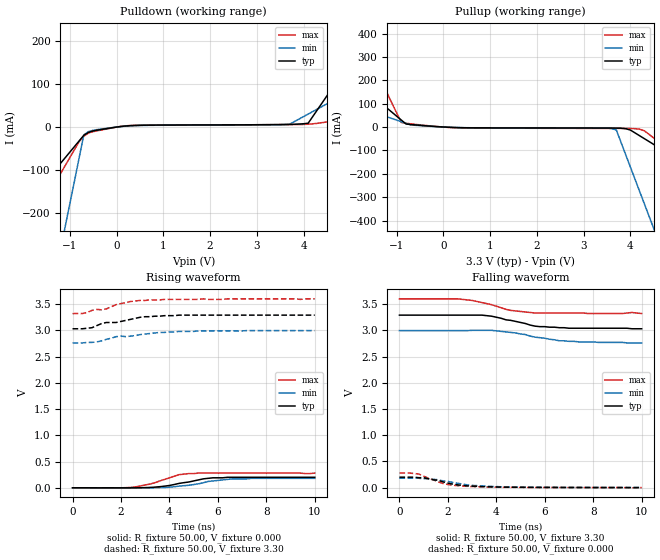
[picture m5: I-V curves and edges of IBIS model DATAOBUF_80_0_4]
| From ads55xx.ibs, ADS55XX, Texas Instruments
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|   Model DATAOBUF_80_0_4
[Model]   DATAOBUF_80_0_4
Model_type   Output
Polarity   Non-Inverting
Vmeas =   1.65V
C_comp   3.00pF   3.00pF   3.00pF
[Temperature Range]   50.00   0.10k   -20.00
[Voltage Range]   3.30V   3.00V   3.60V
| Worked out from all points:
|   slope of the pulldown table from 0 to 0.495 V, typ, clamps not added: 120 ohm
|   slope of the pullup table from 0 to 0.495 V, typ, clamps not added: 147 ohm
|   rising waveform, R_fixture 50.00, V_fixture 0.000: 20-80 % time 1.36ns typ, 1.56ns min, 1.2ns max; typ from 0 V to 0.2 V
|   rising waveform, R_fixture 50.00, V_fixture 3.30: 20-80 % time 1.72ns typ, 2.11ns min, 1.56ns max; typ from 3.03 V to 3.29 V
|   falling waveform, R_fixture 50.00, V_fixture 3.30: 20-80 % time 1.46ns typ, 1.71ns min, 1.42ns max; typ from 3.29 V to 3.03 V
|   falling waveform, R_fixture 50.00, V_fixture 0.000: 20-80 % time 1.35ns typ, 1.57ns min, 1.07ns max; typ from 0.2 V to 0.002 V
[Pulldown]
| voltage   I(typ)   I(min)   I(max)
-3.3V     -359.2mA   -1.41A     -501.7mA
-2.3V     -228.4mA   -874.4mA   -314.5mA
-1.9V     -176.1mA   -660.4mA   -239.6mA
-1.5V     -123.7mA   -446.3mA   -164.7mA
-1V       -58.35mA   -178.7mA   -71.13mA
-700mV    -19.11mA   -18.13mA   -21.33mA
-500mV    -8.95mA    -7.42mA    -10.52mA
300mV     3.33mA     2.8mA      3.59mA
3.7V      6.18mA     6.49mA     5.76mA
4.1V      8.96mA     30.21mA    6.69mA
5.5V      230.9mA    113.2mA    28.31mA
6.6V      405.2mA    178.5mA    46.3mA
[Pullup]
| voltage   I(typ)   I(min)   I(max)
-3.3V     431.1mA    186.7mA    1.012A
-1.9V     197.1mA    91.11mA    432.9mA
-900mV    29.86mA    22.81mA    19mA
-800mV    13.14mA    15.98mA    16.23mA
400mV     -2.71mA    -2.43mA    -3.79mA
3.6V      -4.13mA    -6.27mA    -5.71mA
3.7V      -4.24mA    -12.84mA   -5.75mA
4V        -12.77mA   -170.9mA   -6.09mA
4.2V      -37.39mA   -276.3mA   -9.17mA
4.3V      -49.7mA    -329mA     -16.11mA
4.5V      -74.32mA   -434.4mA   -46.48mA
6.6V      -332.8mA   -1.541A    -365.4mA
[Ramp]
| variable   typ   min   max
dV/dt_r   0.12/1.35n   0.11/1.46n   0.17/1.16n
dV/dt_f   0.16/1.56n   0.14/1.68n   0.16/1.39n
R_load = 50.00
[Rising Waveform]
R_fixture = 50.00
V_fixture = 0.000
V_fixture_min = 0.000
V_fixture_max = 0.000
| time   V(typ)   V(min)   V(max)
0s        19.37nV    23.56nV    42.13nV
2ns       -1.37mV    -180uV     -590uV
2.6ns     -1mV       -1.4mV     16.41mV
3.2ns     6.15mV     -960uV     70.82mV
3.6ns     20.58mV    2.09mV     130mV
4.4ns     83.59mV    31.21mV    250mV
4.8ns     110mV      48.2mV     270mV
5.6ns     180mV      120mV      280mV
6.6ns     200mV      170mV      280mV
10ns      200mV      180mV      280mV
[Rising Waveform]
R_fixture = 50.00
V_fixture = 3.30
V_fixture_min = 3.00
V_fixture_max = 3.60
| time   V(typ)   V(min)   V(max)
0s        3.03V      2.76V      3.32V
400ps     3.03V      2.76V      3.32V
800ps     3.05V      2.77V      3.38V
1.2ns     3.13V      2.8V       3.39V
1.8ns     3.15V      2.88V      3.49V
2.2ns     3.19V      2.88V      3.53V
2.8ns     3.25V      2.92V      3.57V
3.6ns     3.27V      2.96V      3.58V
5.2ns     3.29V      2.99V      3.59V
10ns      3.29V      2.995V     3.6V
[Falling Waveform]
R_fixture = 50.00
V_fixture = 3.30
V_fixture_min = 3.00
V_fixture_max = 3.60
| time   V(typ)   V(min)   V(max)
0s        3.29V      2.995V     3.6V
2.4ns     3.29V      2.995V     3.6V
3.4ns     3.29V      3V         3.53V
4.6ns     3.19V      2.96V      3.38V
5.2ns     3.13V      2.92V      3.35V
5.6ns     3.08V      2.87V      3.33V
6.6ns     3.05V      2.8V       3.33V
9.2ns     3.04V      2.77V      3.32V
9.6ns     3.03V      2.76V      3.34V
10ns      3.03V      2.76V      3.32V
[Falling Waveform]
R_fixture = 50.00
V_fixture = 0.000
V_fixture_min = 0.000
V_fixture_max = 0.000
| time   V(typ)   V(min)   V(max)
0s        200mV      180mV      280mV
400ps     200mV      180mV      280mV
800ps     190mV      180mV      260mV
1ns       190mV      170mV      220mV
1.2ns     170mV      170mV      180mV
1.8ns     110mV      130mV      79.68mV
2.2ns     68.22mV    100mV      47.15mV
2.8ns     34.64mV    53.6mV     25.29mV
4.4ns     9.42mV     14.53mV    6.77mV
10ns      1.8mV      2.16mV     1.45mV
